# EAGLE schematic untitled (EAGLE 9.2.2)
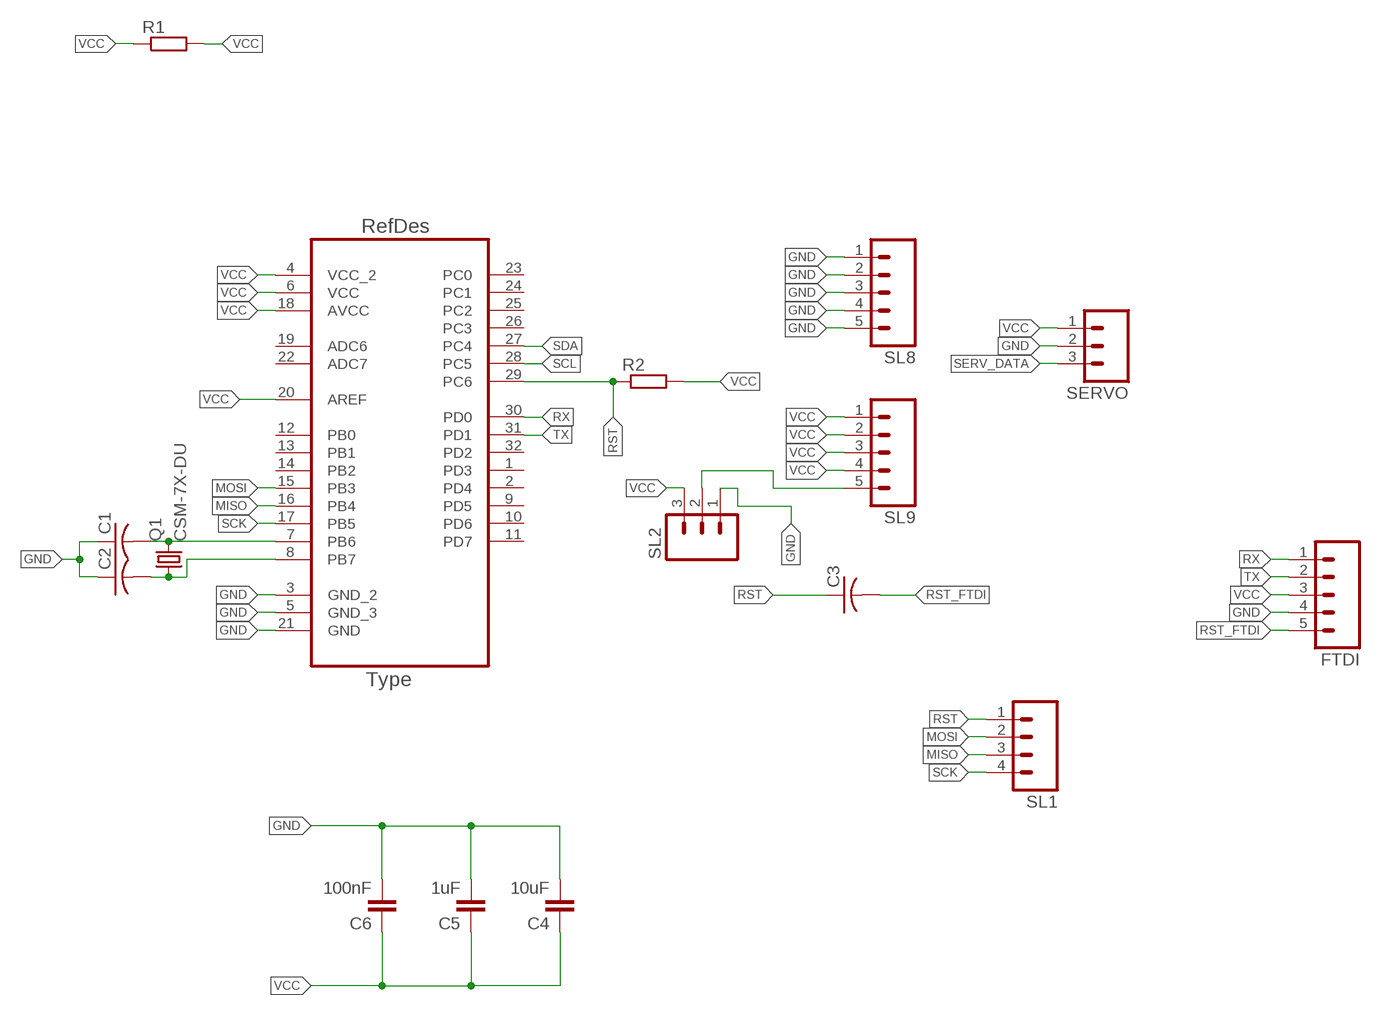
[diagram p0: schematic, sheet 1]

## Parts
C1  C-USC1206  [C1206]
C2  C-USC1206  [C1206]
C3  C-USC1206  [C1206]
C4  10uF  CAP1206  [1206]
C5  1uF  CAP1206  [1206]
C6  100nF  CAP1206  [1206]
FTDI  M05  [05P]
Q1  CSM-7X-DU  [CSM-7X-DU]
R1  RR1206  [R1206]
R2  RR1206  [R1206]
SERVO  M03  [03P]
SL1  M04  [04P]
SL2  M03  [03P]
SL8  M05  [05P]
SL9  M05  [05P]
U1  ATMEGA328P-AU  [QFP80P900X900X120-32N]

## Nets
GND: C1.1 C2.1 C4.2 C5.2 C6.2 FTDI.4 SERVO.2 SL2.1 SL8.1 SL8.2 SL8.3 SL8.4 SL8.5 U1.3(GND_2) U1.5(GND_3) U1.21(GND)
MISO: SL1.3 U1.16(PB4)
MOSI: SL1.2 U1.15(PB3)
N$1: SL2.2 SL9.5
N$2: C1.2 Q1.2 U1.7(PB6)
N$3: C2.2 Q1.1 U1.8(PB7)
RST: C3.1 R2.1 SL1.1 U1.29(PC6)
RST_FTDI: C3.2 FTDI.5
RX: FTDI.1 U1.30(PD0)
SCK: SL1.4 U1.17(PB5)
SCL: U1.28(PC5)
SDA: U1.27(PC4)
SERV_DATA: SERVO.3
TX: FTDI.2 U1.31(PD1)
VCC: C4.1 C5.1 C6.1 FTDI.3 R1.1 R1.2 R2.2 SERVO.1 SL2.3 SL9.1 SL9.2 SL9.3 SL9.4 U1.4(VCC_2) U1.6(VCC) U1.18(AVCC) U1.20(AREF)
Unconnected: U1.1(PD3) U1.2(PD4) U1.9(PD5) U1.10(PD6) U1.11(PD7) U1.12(PB0) U1.13(PB1) U1.14(PB2) U1.19(ADC6) U1.22(ADC7) U1.23(PC0) U1.24(PC1) U1.25(PC2) U1.26(PC3) U1.32(PD2)

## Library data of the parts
C1-C3 = adafruit:C-US: CAPACITOR, American symbol
C4-C6 = 01_SparkFun:CAP: Capacitor
FTDI SL8 SL9 = con-amp-quick:M05: AMP QUICK CONNECTOR; OC_FARNELL: unknown; OC_NEWARK: unknown
Q1 = FAB_Hello:CSM-7X-DU: SMD CRYSTAL; OC_FARNELL: unknown; OC_NEWARK: unknown
R1 R2 = eagle-ltspice:R: RESISTOR, European symbol; SPICEMODEL: NONE; SPICEPREFIX: R
SERVO SL2 = con-amp-quick:M03: AMP QUICK CONNECTOR; OC_FARNELL: unknown; OC_NEWARK: unknown
SL1 = con-amp-quick:M04: AMP QUICK CONNECTOR; OC_FARNELL: unknown; OC_NEWARK: unknown
U1 = Atmel-ATMEGA328P-AU:ATMEGA328P-AU; DESCRIPTION: 8-bit Microcontroller with In-System Programmable Flash; MPN: ATMEGA328P-AU; OC_FARNELL: 1715486; OC_NEWARK: 14R4631; PACKAGE: TQFP-32; SUPPLIER: Atmel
